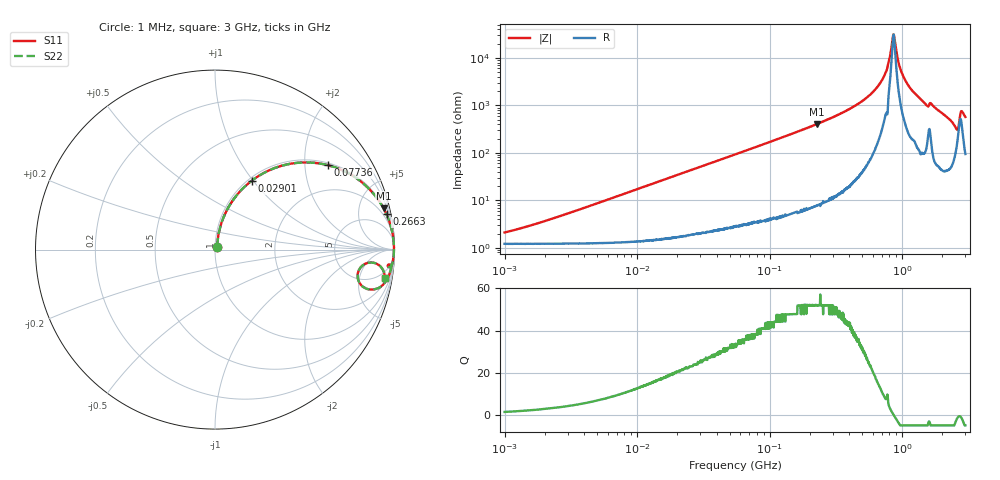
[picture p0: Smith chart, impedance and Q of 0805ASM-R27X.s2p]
!s-Parameter Generated by FASTRON Sdn. Bhd.
!FASTRON P/N : 0805ASM-R27X
!Keysight Technologies: E4991B_MY54100416_A.01.15
!Date: Fri Jun 19 14:51:39 2026
!Version  :Rev00  Fri Jun 19 14:51:39 2026
!Data & Calibration Information:
!Freq  S11  S21  S12  S22
!PortZ  Port1:50+j0  Port2:50+j0
!When reading reference impedance value at option line is always used.
! Remarks : This data is being provided solely for informational purposes.
# Hz S dB R 50
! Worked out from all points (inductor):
!   1601 points, 1 MHz to 3 GHz, reference 50 ohm
!   read as one part in series: L = 273 nH near 2.14 MHz
!   highest Q = 52.1 at 228 MHz (marker M1), where L = 284 nH
!   self-resonance near 858.7 MHz
!   S11 on the Smith chart (normalised r, x): 1 MHz: 1.02, +0.03; 29.01 MHz: 1.04, +0.98; 77.36 MHz: 1.07, +2.61; 266.3 MHz: 1.18, +9.70; 3 GHz: 3, -11
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1000000  -33.60 53.8  -0.11 -1.0  -0.11 -1.0  -33.60 53.8
3804036  -23.70 75.6  -0.12 -3.7  -0.12 -3.7  -23.70 75.6
1.447069e7  -12.50 72.9  -0.38 -13.7  -0.38 -13.7  -12.50 72.9
2.90111e7  -7.23 61.9  -1.08 -25.8  -1.08 -25.8  -7.23 61.9
5.504702e7  -3.47 46.2  -2.83 -42.1  -2.83 -42.1  -3.47 46.2
7.735911e7  -2.11 36.9  -4.43 -51.6  -4.43 -51.6  -2.11 36.9
2.083556e8  -0.35 15.2  -11.60 -73.7  -11.60 -73.7  -0.35 15.2
2.279937e8  -0.29 13.8  -12.50 -75.1  -12.50 -75.1  -0.29 13.8
2.662515e8  -0.21 11.6  -14.00 -77.3  -14.00 -77.3  -0.21 11.6
5.840965e8  -0.04 3.2  -25.00 -84.2  -25.00 -84.2  -0.04 3.2
7.135306e8  -0.03 1.6  -31.30 -82.8  -31.30 -82.8  -0.03 1.6
7.925923e8  -0.02 0.7  -38.60 -76.8  -38.60 -76.8  -0.02 0.7
8.374426e8  -0.03 0.2  -46.10 -52.7  -46.10 -52.7  -0.03 0.2
8.672962e8  -0.03 -0.1  -49.60 15.5  -49.60 15.5  -0.03 -0.1
9.977393e8  -0.03 -1.2  -33.50 79.8  -33.50 79.8  -0.03 -1.2
1.237271e9  -0.06 -3.1  -25.30 81.4  -25.30 81.4  -0.06 -3.1
1.511446e9  -0.13 -5.4  -20.50 78.3  -20.50 78.3  -0.13 -5.4
1.67054e9  -0.14 -5.3  -20.60 77.7  -20.60 77.7  -0.14 -5.3
2.156205e9  -0.23 -9.6  -15.50 76.2  -15.50 76.2  -0.23 -9.6
2.530652e9  -0.99 -14.4  -11.70 58.6  -11.70 58.6  -0.99 -14.4
2.811057e9  -0.64 -5.9  -18.20 51.7  -18.20 51.7  -0.64 -5.9
3e9  -0.37 -9.6  -15.50 70.9  -15.50 70.9  -0.37 -9.6
